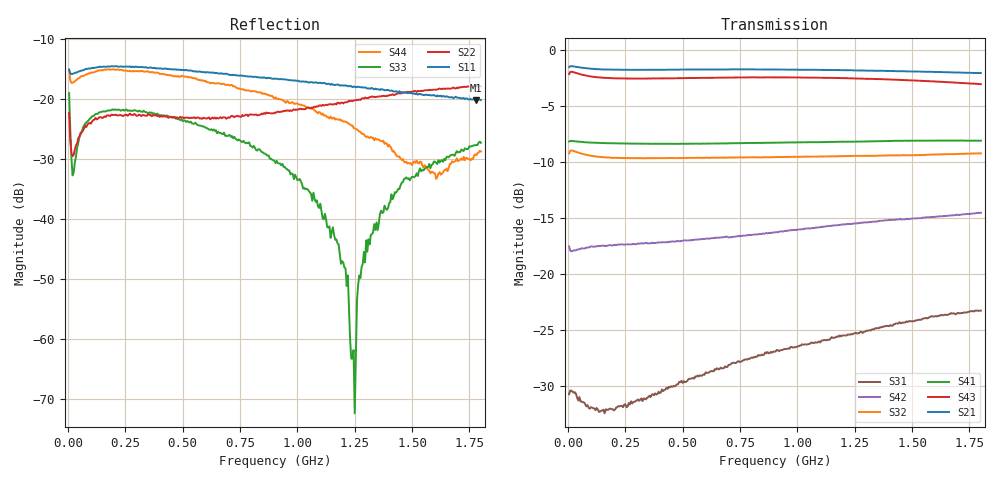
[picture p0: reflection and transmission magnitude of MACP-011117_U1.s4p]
!Agilent Technologies,E5071C,MY46630996,B.13.30
!Date: Tue Jan 23 09:24:13 2024
!Data & Calibration Information:
!MACP-011117 soldered onto PT-0013779 with F connectors, Calibration PT-0003645-TRL. Port1 (pin1) Port2 (pin5) Port3 (pin4) Port4 (pin3)
!Freq	S11:SOLT4(ON)	S12:SOLT4(ON)	S13:SOLT4(ON)	S14:SOLT4(ON)
!	S21:SOLT4(ON)	S22:SOLT4(ON)	S23:SOLT4(ON)	S24:SOLT4(ON)
!	S31:SOLT4(ON)	S32:SOLT4(ON)	S33:SOLT4(ON)	S34:SOLT4(ON)
!	S41:SOLT4(ON)	S42:SOLT4(ON)	S43:SOLT4(ON)	S44:SOLT4(ON)
!PortZ  Port1:75+j0  Port2:75+j0  Port3:75+j0  Port4:75+j0
!Above PortZ is port z conversion or system Z0 setting when saving the data.
!When reading, reference impedance value at option line is always used.
# Hz S MA R 75
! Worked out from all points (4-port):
!   360 points, 5 MHz to 1.8 GHz, reference 75 ohm
!   strongest paths, dB at 5 MHz, 455 MHz, 905 MHz, 1.355 GHz, 1.8 GHz:
!     S21: -1.5, -1.7, -1.7, -1.8, -2.1
!     S43: -2.1, -2.5, -2.4, -2.6, -3.0
!     S41: -8.2, -8.4, -8.3, -8.1, -8.1
!     S32: -9.2, -9.6, -9.5, -9.4, -9.2
!     S42: -17.5, -17.1, -16.3, -15.3, -14.5
!     S31: -30.7, -30.0, -26.9, -24.8, -23.2
!   lowest |S11| = -20.2 dB at 1.78 GHz (marker M1), VSWR 1.22, Z = 61.7 + j1.69 ohm
!   |S11| at or under -10 dB: start of sweep to end of sweep
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5000000  0.1769 165.5  0.8389 3.1  0.02951 20.5  0.3908 -178.5
         0.8403 3.3  0.07691 127.8  0.3453 7.2  0.134 173.5
         0.02918 17.4  0.3466 7.1  0.1124 116.2  0.781 5.7
         0.391 -178.6  0.133 174.0  0.782 5.7  0.1758 155.4
1.07e9  0.1374 168.9  0.8172 -18.9  0.04656 15.3  0.3874 118.7
        0.8174 -18.9  0.08572 -136.1  0.3348 -9.5  0.1628 129.4
        0.04948 16.5  0.3347 -9.3  0.01662 159.6  0.7534 -33.5
        0.3884 118.8  0.1606 128.3  0.7535 -33.5  0.08275 97.3
1.22e9  0.1289 169.4  0.8122 -21.7  0.05048 12.4  0.3895 110.5
        0.8131 -21.7  0.09519 -132.7  0.3368 -10.9  0.1693 121.6
        0.05388 13.0  0.3368 -10.8  0.003399 -178.9  0.7486 -38.9
        0.3904 110.6  0.1674 120.5  0.7488 -38.9  0.06328 83.1
1.25e9  0.1271 169.2  0.8113 -22.3  0.0513 11.0  0.3896 108.8
        0.8119 -22.3  0.09774 -132.0  0.3374 -11.2  0.17 120.1
        0.05453 12.3  0.3371 -11.2  0.0002407 26.1  0.7472 -40.0
        0.3906 109.0  0.1686 119.0  0.7474 -40.0  0.05716 80.9
1.3e9  0.1246 169.7  0.8093 -23.2  0.05212 10.0  0.3897 106.1
       0.8101 -23.2  0.1023 -131.0  0.3375 -11.7  0.1716 117.6
       0.05598 11.3  0.3371 -11.7  0.006659 -36.3  0.7449 -41.8
       0.3915 106.4  0.1704 116.5  0.7449 -41.8  0.04847 71.6
1.78e9  0.0982 172.1  0.7896 -31.7  0.06322 -6.5  0.3923 80.4
        0.7903 -31.9  0.1278 -131.3  0.3456 -17.1  0.1902 95.2
        0.06879 -6.1  0.3461 -16.9  0.04144 -39.9  0.7068 -60.1
        0.3947 80.4  0.1877 93.7  0.7071 -60.1  0.03417 -55.4
1.8e9  0.09835 171.0  0.7893 -32.1  0.06345 -7.3  0.392 79.3
       0.7897 -32.3  0.1283 -131.7  0.3458 -17.3  0.1908 94.2
       0.06888 -6.6  0.3463 -17.2  0.04329 -40.0  0.7042 -60.9
       0.3943 79.3  0.188 92.9  0.705 -60.9  0.03666 -60.4
